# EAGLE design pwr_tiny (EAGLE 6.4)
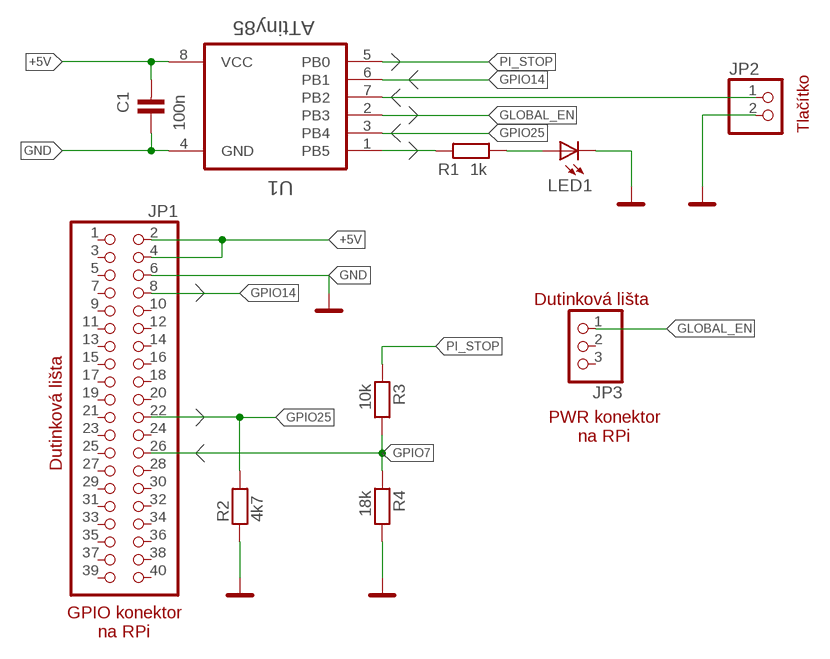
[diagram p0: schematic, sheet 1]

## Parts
C1  100n  C-KERAMIK_SMD_1206  [1206]
JP1  PINHD-2X20  [2X20]
JP2  PINHD-1X2  [1X02]
JP3  PINHD-1X3  [1X03]
LED1  LED3MM  [LED3MM]
R1  1k  R_SMD_0805  [0805]
R2  4k7  R_SMD_0805  [0805]
R3  10k  R_SMD_0805  [0805]
R4  18k  R_SMD_0805  [0805]
U1  ATtiny85  ATTINY85-20PU  [DIP254P762X533-8]

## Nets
+5V: C1.2 JP1.2 JP1.4 U1.8(VCC)
GLOBAL_EN: JP3.1 U1.2(PB3)
GND: C1.1 JP1.6 JP2.2 LED1.K(C) R2.1 R4.2 U1.4(GND)
GPIO7: JP1.26 R3.2 R4.1
GPIO14: JP1.8 U1.6(PB1)
GPIO25: JP1.22 R2.2 U1.3(PB4)
LED-INFO: LED1.A R1.1
PB2-TLACITKO: JP2.1 U1.7(PB2)
PB5-INFOLED: R1.2 U1.1(PB5)
PI_STOP: R3.1 U1.5(PB0)
Unconnected: JP1.1 JP1.3 JP1.5 JP1.7 JP1.9 JP1.10 JP1.11 JP1.12 JP1.13 JP1.14 JP1.15 JP1.16 JP1.17 JP1.18 JP1.19 JP1.20 JP1.21 JP1.23 JP1.24 JP1.25 JP1.27 JP1.28 JP1.29 JP1.30 JP1.31 JP1.32 JP1.33 JP1.34 JP1.35 JP1.36 JP1.37 JP1.38 JP1.39 JP1.40 JP3.2 JP3.3

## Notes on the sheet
- Tlačítko
- Dutinková lišta
- PWR konektor
  na RPi
- Dutinková lišta
- GPIO konektor
  na RPi

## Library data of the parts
C1 = #PaJa_30:C-KERAMIK: Kondenzator - keramicky
JP1 = dut_lista:PINHD-2X20: PIN HEADER
JP2 = pinhead:PINHD-1X2: PIN HEADER
JP3 = dut_lista:PINHD-1X3: PIN HEADER
LED1 = adafruit:LED: LED
R1-R4 = #PaJa_30:R: Rezistor
U1 = Atmel_By_element14_Batch_1-00:ATTINY85-20PU: 8-bit Microcontroller with In-System Programmable Flash; MPN: ATTINY85-20PU; OC_FARNELL: 1455162; OC_NEWARK: 58M3796; PACKAGE: PDIP-8; SUPPLIER: Atmel

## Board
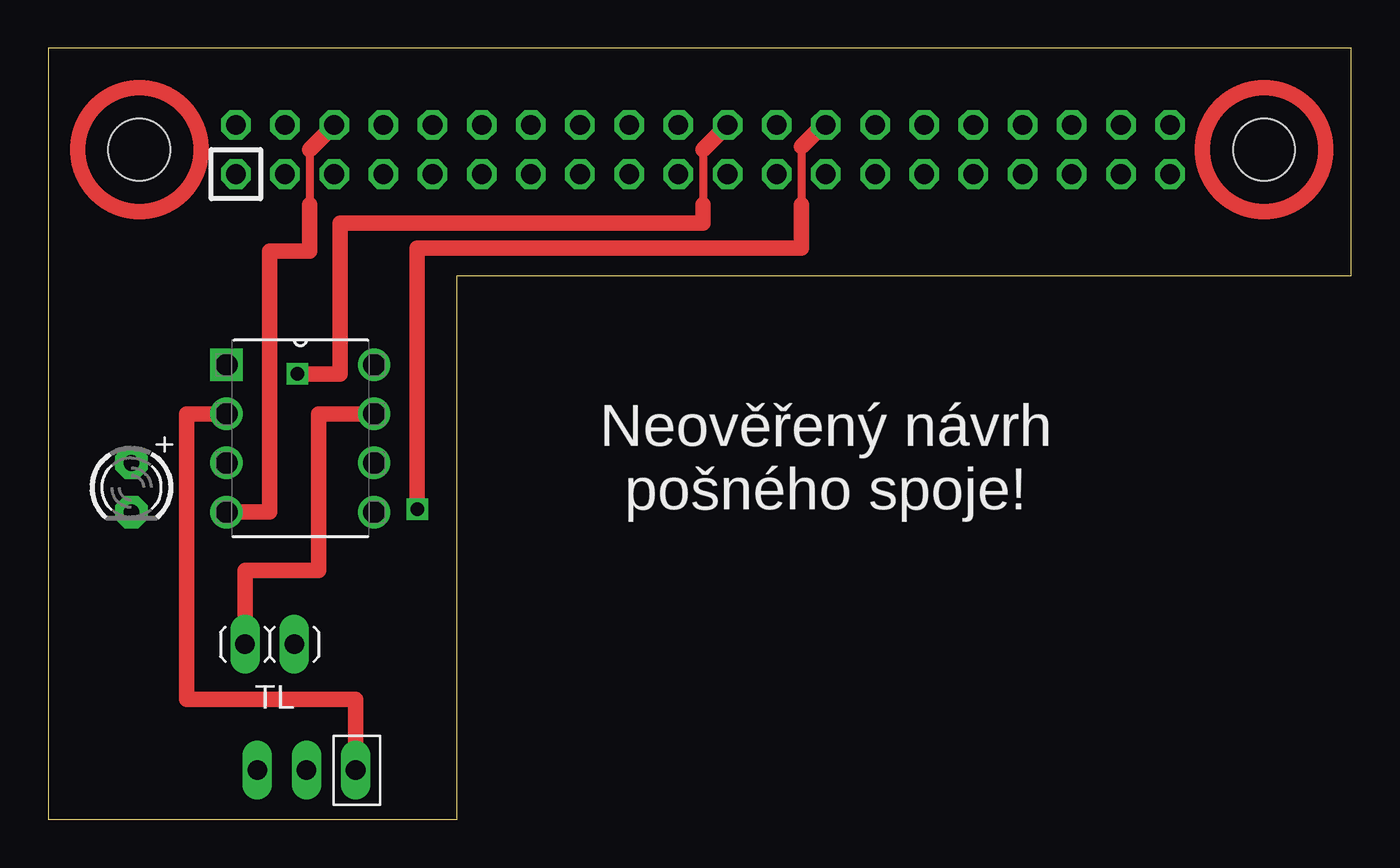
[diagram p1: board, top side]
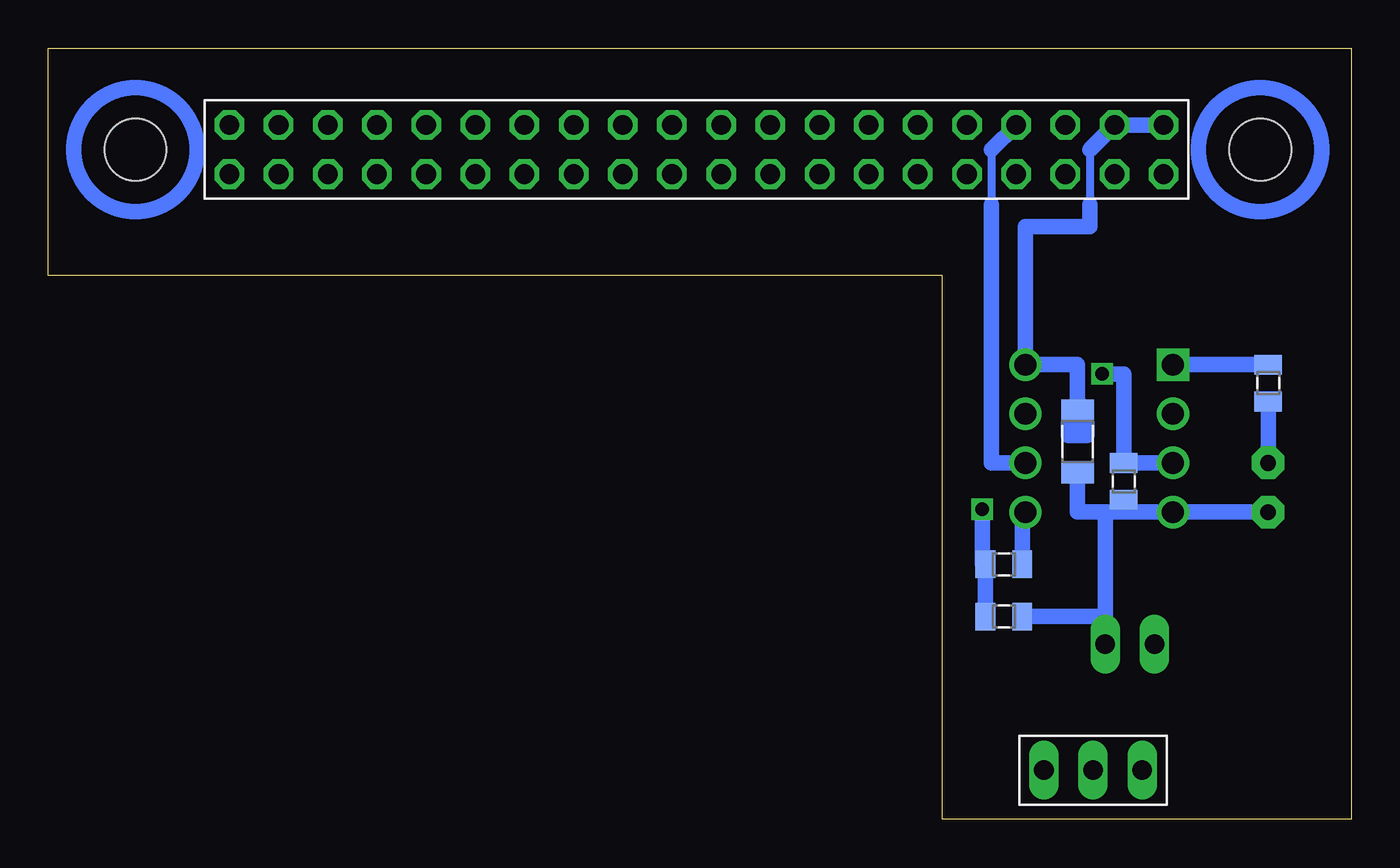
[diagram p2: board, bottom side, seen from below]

Size 67.3 x 39.84 mm. Coordinates in mm from the lower left corner, seen from the top.
Outline: 0,0 21.11,0 21.11,28.1 67.3,28.1 67.3,39.84 0,39.84 0,0
Copper layers (1*16): Top 0.035mm / dielectric 1.5mm / Bottom 0.035mm
Design rules "default *": minimum track width 10mil, minimum drill 24mil, track to track 8mil, track to pad 8mil, pad to pad 8mil, via to via 8mil, smd to smd 8mil, copper to edge 40mil, drill to drill 8mil, minimum pad ring 10mil, minimum via ring 8mil, stop-mask expansion 4mil, vias tented up to drill 0mil, thermal gap 10mil
Holes 3.2 mm at 62.8,34.61 4.7,34.61

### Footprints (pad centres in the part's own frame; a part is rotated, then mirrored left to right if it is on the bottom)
1206 = smd 1.143 x 1.702: 1 -1.587,0; 2 1.587,0
2X20 = drill 1.016 octagon: 1 -24.13,1.27; 2 -24.13,-1.27; 3 -21.59,1.27; 4 -21.59,-1.27; 5 -19.05,1.27; 6 -19.05,-1.27; 7 -16.51,1.27; 8 -16.51,-1.27; 9 -13.97,1.27; 10 -13.97,-1.27; 11 -11.43,1.27; 12 -11.43,-1.27; 13 -8.89,1.27; 14 -8.89,-1.27; 15 -6.35,1.27; 16 -6.35,-1.27; 17 -3.81,1.27; 18 -3.81,-1.27; 19 -1.27,1.27; 20 -1.27,-1.27; 21 1.27,1.27; 22 1.27,-1.27; 23 3.81,1.27; 24 3.81,-1.27; 25 6.35,1.27; 26 6.35,-1.27; 27 8.89,1.27; 28 8.89,-1.27; 29 11.43,1.27; 30 11.43,-1.27; 31 13.97,1.27; 32 13.97,-1.27; 33 16.51,1.27; 34 16.51,-1.27; 35 19.05,1.27; 36 19.05,-1.27; 37 21.59,1.27; 38 21.59,-1.27; 39 24.13,1.27; 40 24.13,-1.27
1X02 = drill 1.016 long: 1 -1.27,0; 2 1.27,0
1X03 = drill 1.016 long: 1 2.54,0; 2 0,0; 3 -2.54,0
LED3MM = drill 0.813 pad 1.676 octagon: A -1.27,0; K 1.27,0
0805 = smd 1.016 x 1.422: 1 -0.953,0; 2 0.953,0
DIP254P762X533-8 = drill 1.118 square: 1 -7.62,7.62 | drill 1.118: 2 -7.62,5.08; 3 -7.62,2.54; 4 -7.62,0; 5 0,0; 6 0,2.54; 7 0,5.08; 8 0,7.62

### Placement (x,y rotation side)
C1  14.13,19.53 90 bottom
JP1  33.81,34.61 180 bottom
JP2  11.43,9.05 0 top
JP3  13.34,2.54 180 bottom
LED1  4.29,17.14 270 top
R1  4.29,22.54 90 bottom
R2  11.75,17.46 90 bottom
R3  17.94,13.18 180 bottom
R4  17.94,10.48 0 bottom
U1  16.83,15.88 0 top

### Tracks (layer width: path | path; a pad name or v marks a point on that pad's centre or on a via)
+5V
  Bottom 0.406: 13.49,34.61 13.49,31.75
  Bottom 0.813: JP1.2 JP1.4 13.49,34.61 | 13.49,31.75 13.49,30.64 16.83,30.64 U1.8 14.13,23.5 C1.2
GLOBAL_EN
  Top 0.813: U1.2 7.14,20.96 7.14,6.19 15.88,6.19 JP3.1
GND
  Top 0.406: 13.49,34.61 13.49,31.75
  Top 0.813: JP1.6 13.49,34.61 | 13.49,31.75 13.49,29.37 11.43,29.37 11.43,15.88 U1.4
  Bottom 0.813: R4.2 12.7,10.48 | 12.7,10.48 JP2.2 | LED1.K U1.4 11.75,15.88 | C1.1 14.13,15.88 12.7,15.88 | 12.7,15.88 11.75,15.88 | R2.1 11.75,15.88 | 12.7,10.48 12.7,15.88
GPIO7  (via drill 0.7)
  Top 0.406: 38.89,34.77 38.89,31.75
  Top 0.813: v19.05,16.03 19.05,29.53 38.89,29.53 38.89,31.75 | JP1.26 40.01,35.88 38.89,34.77
  Bottom 0.813: R4.1 R3.2 19.05,13.18 v19.05,16.03
GPIO14
  Bottom 0.406: 18.57,34.61 18.57,31.75
  Bottom 0.813: JP1.8 18.57,34.61 | 18.57,31.75 18.57,18.42 U1.6
GPIO25  (via drill 0.7)
  Top 0.406: 33.81,34.61 33.81,31.75
  Top 0.813: JP1.22 33.81,34.61 | 33.81,31.75 33.81,30.8 15.08,30.8 15.08,23.02 v12.86,23.02
  Bottom 0.813: U1.3 R2.2 11.75,23.02 v12.86,23.02
LED-INFO
  Bottom 0.813: R1.1 LED1.A
N$1
  Bottom 0.813: 13.65,19.84 13.65,20.48 14.61,20.48 14.61,19.84 13.65,19.84
PB2-TLACITKO
  Top 0.813: JP2.1 10.16,12.86 13.97,12.86 13.97,20.96 U1.7
PB5-INFOLED
  Bottom 0.813: U1.1 R1.2
PI_STOP
  Bottom 0.813: U1.5 16.99,15.88 R3.1
(copper drawn outside any net)
  shapes: Bottom circle x2, Top circle x2

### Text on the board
tPlace: Neověřený návrh / pošného spoje! | TL
tDocu: Global_EN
